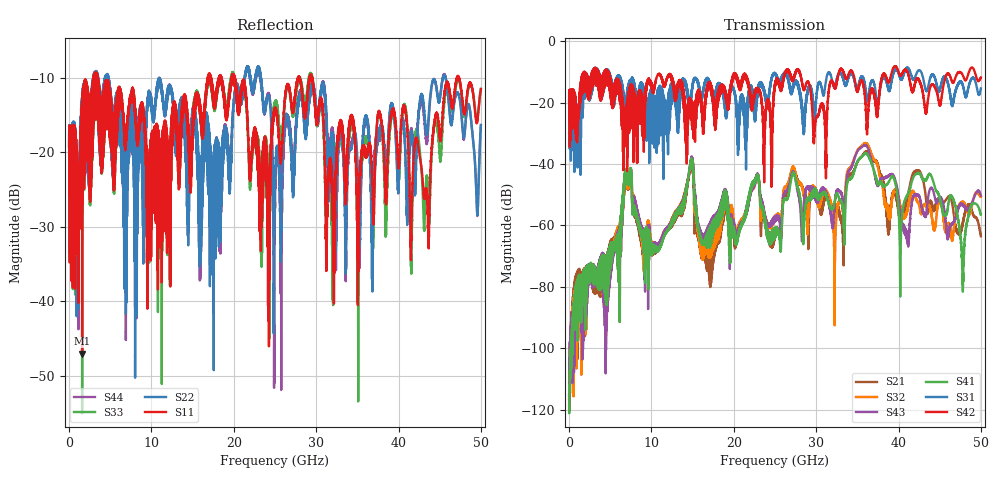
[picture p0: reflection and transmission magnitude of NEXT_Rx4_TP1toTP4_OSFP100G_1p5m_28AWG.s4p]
! Touchstone data
! Created: 27-Feb-2019 by IdEM 12 (12.1.0)
! COMMENTS
!  Created Wed Feb 27 09:43:39 2019
!  64 Port Network Data from SP1.SP block
!  freq  magS1_1  angS1_1  magS1_2  angS1_2  magS1_3  angS1_3  magS1_4  angS1_4
!  magS1_5  angS1_5  magS1_6  angS1_6  magS1_7  angS1_7  magS1_8  angS1_8
!  magS1_9  angS1_9  magS1_10  angS1_10  magS1_11  angS1_11  magS1_12  angS1_12
!  magS1_13  angS1_13  magS1_14  angS1_14  magS1_15  angS1_15  magS1_16  angS1_16
!  magS1_17  angS1_17  magS1_18  angS1_18  magS1_19  angS1_19  magS1_20  angS1_20
!  magS1_21  angS1_21  magS1_22  angS1_22  magS1_23  angS1_23  magS1_24  angS1_24
!  magS1_25  angS1_25  magS1_26  angS1_26  magS1_27  angS1_27  magS1_28  angS1_28
!  magS1_29  angS1_29  magS1_30  angS1_30  magS1_31  angS1_31  magS1_32  angS1_32
!  magS1_33  angS1_33  magS1_34  angS1_34  magS1_35  angS1_35  magS1_36  angS1_36
!  magS1_37  angS1_37  magS1_38  angS1_38  magS1_39  angS1_39  magS1_40  angS1_40
!  magS1_41  angS1_41  magS1_42  angS1_42  magS1_43  angS1_43  magS1_44  angS1_44
!  magS1_45  angS1_45  magS1_46  angS1_46  magS1_47  angS1_47  magS1_48  angS1_48
!  magS1_49  angS1_49  magS1_50  angS1_50  magS1_51  angS1_51  magS1_52  angS1_52
!  magS1_53  angS1_53  magS1_54  angS1_54  magS1_55  angS1_55  magS1_56  angS1_56
!  magS1_57  angS1_57  magS1_58  angS1_58  magS1_59  angS1_59  magS1_60  angS1_60
!  magS1_61  angS1_61  magS1_62  angS1_62  magS1_63  angS1_63  magS1_64  angS1_64
!  magS2_1  angS2_1  magS2_2  angS2_2  magS2_3  angS2_3  magS2_4  angS2_4
!  magS2_5  angS2_5  magS2_6  angS2_6  magS2_7  angS2_7  magS2_8  angS2_8
!  magS2_9  angS2_9  magS2_10  angS2_10  magS2_11  angS2_11  magS2_12  angS2_12
!  magS2_13  angS2_13  magS2_14  angS2_14  magS2_15  angS2_15  magS2_16  angS2_16
!  magS2_17  angS2_17  magS2_18  angS2_18  magS2_19  angS2_19  magS2_20  angS2_20
!  magS2_21  angS2_21  magS2_22  angS2_22  magS2_23  angS2_23  magS2_24  angS2_24
!  magS2_25  angS2_25  magS2_26  angS2_26  magS2_27  angS2_27  magS2_28  angS2_28
!  magS2_29  angS2_29  magS2_30  angS2_30  magS2_31  angS2_31  magS2_32  angS2_32
!  magS2_33  angS2_33  magS2_34  angS2_34  magS2_35  angS2_35  magS2_36  angS2_36
!  magS2_37  angS2_37  magS2_38  angS2_38  magS2_39  angS2_39  magS2_40  angS2_40
!  magS2_41  angS2_41  magS2_42  angS2_42  magS2_43  angS2_43  magS2_44  angS2_44
!  magS2_45  angS2_45  magS2_46  angS2_46  magS2_47  angS2_47  magS2_48  angS2_48
!  magS2_49  angS2_49  magS2_50  angS2_50  magS2_51  angS2_51  magS2_52  angS2_52
!  magS2_53  angS2_53  magS2_54  angS2_54  magS2_55  angS2_55  magS2_56  angS2_56
!  magS2_57  angS2_57  magS2_58  angS2_58  magS2_59  angS2_59  magS2_60  angS2_60
!  magS2_61  angS2_61  magS2_62  angS2_62  magS2_63  angS2_63  magS2_64  angS2_64
!  magS3_1  angS3_1  magS3_2  angS3_2  magS3_3  angS3_3  magS3_4  angS3_4
!  magS3_5  angS3_5  magS3_6  angS3_6  magS3_7  angS3_7  magS3_8  angS3_8
!  magS3_9  angS3_9  magS3_10  angS3_10  magS3_11  angS3_11  magS3_12  angS3_12
!  magS3_13  angS3_13  magS3_14  angS3_14  magS3_15  angS3_15  magS3_16  angS3_16
!  magS3_17  angS3_17  magS3_18  angS3_18  magS3_19  angS3_19  magS3_20  angS3_20
!  magS3_21  angS3_21  magS3_22  angS3_22  magS3_23  angS3_23  magS3_24  angS3_24
!  magS3_25  angS3_25  magS3_26  angS3_26  magS3_27  angS3_27  magS3_28  angS3_28
!  magS3_29  angS3_29  magS3_30  angS3_30  magS3_31  angS3_31  magS3_32  angS3_32
!  magS3_33  angS3_33  magS3_34  angS3_34  magS3_35  angS3_35  magS3_36  angS3_36
!  magS3_37  angS3_37  magS3_38  angS3_38  magS3_39  angS3_39  magS3_40  angS3_40
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# Hz S MA R 50
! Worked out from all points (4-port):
!   5000 points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, 10 MHz to 50 GHz, reference 50 ohm
!   strongest paths, dB at 10 MHz, 12.51 GHz, 25.01 GHz, 37.51 GHz, 50 GHz:
!     S42: -19.6, -12.6, -13.6, -21.6, -11.9
!     S31: -19.6, -16.2, -10.8, -21.0, -15.4
!     S41: -118.3, -59.7, -64.1, -46.0, -56.5
!     S43: -115.1, -59.1, -58.8, -46.6, -50.2
!     S32: -115.0, -59.4, -57.8, -41.1, -50.7
!     S21: -116.5, -60.3, -63.8, -40.3, -63.5
!   lowest |S11| = -47.1 dB at 1.59 GHz (marker M1), VSWR 1.01, Z = 49.7 + j0.298 ohm
!   |S11| at or under -10 dB: 3.482 GHz to 16.85 GHz (13.37 GHz wide, 132 % of centre); 20.15 GHz to 27.79 GHz (7.635 GHz wide, 31.9 % of centre); 29.53 GHz to 47.08 GHz (17.55 GHz wide, 45.8 % of centre)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
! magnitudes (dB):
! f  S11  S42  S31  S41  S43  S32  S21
! 10 MHz  -19.2  -19.6  -19.6  -118.3  -115.1  -115.0  -116.5
! 1.59 GHz  -47.1  -17.0  -24.2  -86.4  -101.1  -94.0  -83.4
! 14.81 GHz  -24.7  -19.9  -18.6  -38.7  -38.2  -38.5  -38.9
! 16.32 GHz  -15.3  -29.8  -16.0  -66.1  -64.5  -68.0  -70.5
! 36.08 GHz  -20.6  -25.6  -17.5  -36.5  -34.0  -33.2  -35.9
! 41.04 GHz  -16.4  -9.8  -8.7  -50.4  -64.9  -55.5  -51.4
! 50 GHz  -11.5  -11.9  -15.4  -56.5  -50.2  -50.7  -63.5
